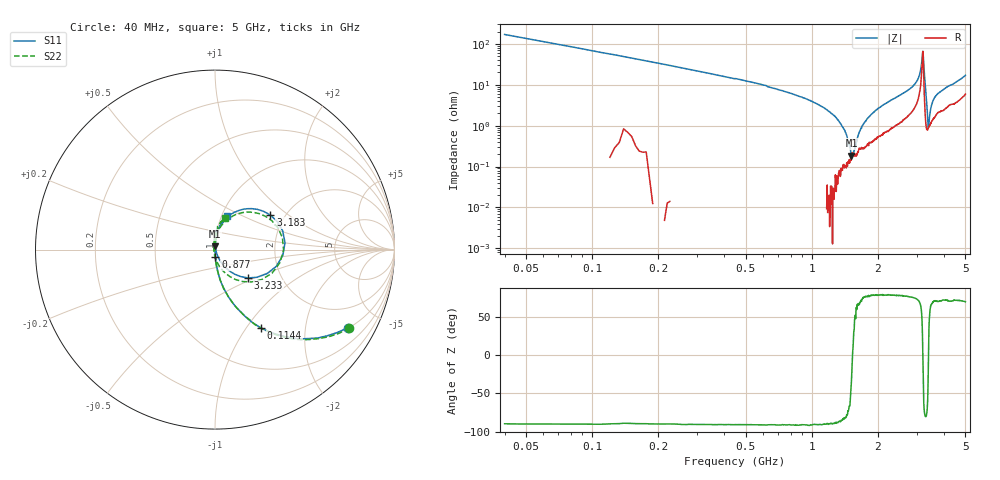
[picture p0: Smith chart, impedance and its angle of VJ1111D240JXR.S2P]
! VJ1111D240JXR
! DATE 02/16/2022  10:18
! CAPACITORS MOUNTED IN SERIES ON 25 MIL THICK MICROSTRIP SUBSTRATE
# GHz  S  MA  R  50.00
!  FREQ  S11M  S11A  S21M  S21A  S12M  S12A  S22M  S22A
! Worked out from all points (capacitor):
!   801 points, 40 MHz to 5 GHz, reference 50 ohm
!   read as one part in series: C = 23.2 pF near 64.8 MHz
!   lowest |Z| = 186 mohm at 1.516 GHz (marker M1)
!   series resonance near 1.533 GHz, so ESL is about 460 pH
!   S11 on the Smith chart (normalised r, x): 40 MHz: 1.02, -3.39; 114.4 MHz: 1.00, -1.18; 877 MHz: 1.00, -0.08; 3.183 GHz: 1.68, +0.75; 3.233 GHz: 1.36, -0.46; 5 GHz: 1.06, +0.41
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0.04  0.8587 -30.5  0.508 59.3  0.5058 59.4  0.8671 -30.3
0.1144  0.5068 -59.5  0.8581 30.8  0.8661 30.6  0.5124 -59.3
0.3004  0.21 -77.7  0.9769 12.5  0.9831 12.3  0.2118 -78.0
0.8708  0.04214 -87.2  0.9991 3.6  1.004 3.5  0.04262 -87.4
0.877  0.04168 -86.8  0.9985 3.6  1.004 3.4  0.04181 -87.5
1.1622  0.0117 -85.5  0.9978 2.3  1.003 2.2  0.01146 -88.2
1.2428  0.004086 -81.3  0.9973 2.0  1.003 1.8  0.004737 -87.2
1.2738  0.002261 -70.7  0.9966 1.9  1.003 1.8  0.001898 -96.5
1.2924  0.0006298 -35.8  0.9971 1.9  1.002 1.7  6.439e-05 -30.3
1.373  0.007091 85.1  0.9962 1.6  1.002 1.4  0.006651 86.0
1.5156  0.01775 86.7  0.9955 1.2  1.001 1.0  0.01702 86.6
1.6954  0.0297 87.2  0.9929 0.7  0.9987 0.5  0.02933 86.8
2.52  0.08263 83.6  0.9777 -1.3  0.9834 -1.5  0.0825 83.4
3.0036  0.1462 75.9  0.9473 -4.3  0.9519 -4.5  0.1447 74.0
3.1834  0.3635 32.0  0.6768 -9.1  0.681 -9.2  0.3551 27.0
3.233  0.2425 -40.6  0.843 16.4  0.8477 16.4  0.2358 -49.0
3.3198  0.01136 -56.8  0.9784 4.9  0.9842 4.7  0.01252 -118.2
3.3508  0.01553 79.7  0.9803 3.5  0.9855 3.3  0.01439 118.3
3.4004  0.03959 87.4  0.9768 2.1  0.9822 2.0  0.03674 100.2
3.5182  0.07093 87.9  0.9695 0.5  0.9749 0.4  0.06318 92.7
4.1754  0.1345 78.1  0.9526 -2.3  0.9571 -2.4  0.1164 79.9
5  0.1968 70.7  0.9114 -5.8  0.9169 -6.0  0.1869 72.6
